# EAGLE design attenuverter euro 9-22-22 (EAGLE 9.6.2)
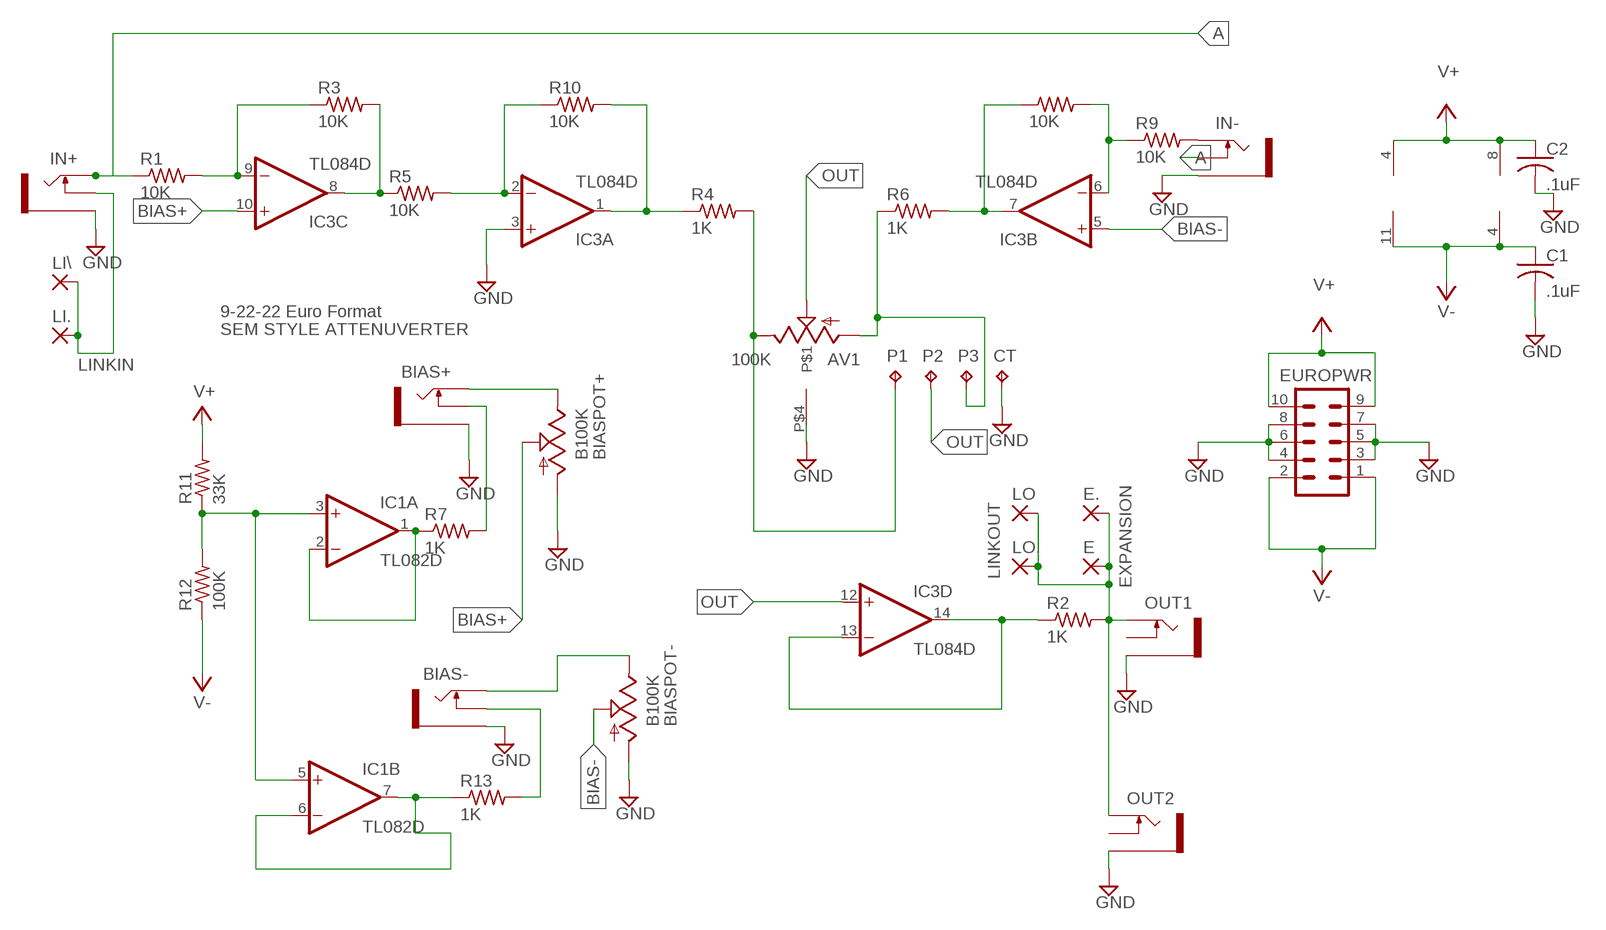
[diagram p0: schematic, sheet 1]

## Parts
AV1  100K  ALPSRK11K114  [ALPSCENTERTAP]
BIAS+  THONKICONNNEW  [WQP-PJ301M-12_JACK]
BIAS-  THONKICONNNEW  [WQP-PJ301M-12_JACK]
BIASPOT+  B100K  9MM_SNAP-IN_POT_  [9MM_SNAP-IN_POT]
BIASPOT-  B100K  9MM_SNAP-IN_POT_  [9MM_SNAP-IN_POT]
C1  .1uF  C-US025-030X050  [C025-030X050]
C2  .1uF  C-US025-030X050  [C025-030X050]
CT  TPPAD1-13  [P1-13]
E  WIREPAD_WIREPAD1,6/0,9  [WIREPAD_1,6/0,9]
E.  WIREPAD_WIREPAD1,6/0,9  [WIREPAD_1,6/0,9]
EUROPWR  EURO_POWER_HEADERREGULAR  [EURO_POWER_HEADER]
IC1  TL082D  [SO08]
IC3  TL084D  [SO14]
IN+  THONKICONNNEW  [WQP-PJ301M-12_JACK]
IN-  THONKICONNNEW  [WQP-PJ301M-12_JACK]
LI.  WIREPAD_WIREPAD1,6/0,9  [WIREPAD_1,6/0,9]
LI\  WIREPAD_WIREPAD1,6/0,9  [WIREPAD_1,6/0,9]
LO  WIREPAD_WIREPAD1,6/0,9  [WIREPAD_1,6/0,9]
LO.  WIREPAD_WIREPAD1,6/0,9  [WIREPAD_1,6/0,9]
OUT1  THONKICONNNEW  [WQP-PJ301M-12_JACK]
OUT2  THONKICONNNEW  [WQP-PJ301M-12_JACK]
P1  TPPAD1-13  [P1-13]
P2  TPPAD1-13  [P1-13]
P3  TPPAD1-13  [P1-13]
R1  10K  R-US_0204/7  [0204/7]
R2  1K  R-US_0204/7  [0204/7]
R3  10K  R-US_0204/7  [0204/7]
R4  1K  R-US_0204/7  [0204/7]
R5  10K  R-US_0204/7  [0204/7]
R6  1K  R-US_0204/7  [0204/7]
R7  1K  R-US_0204/7  [0204/7]
R8  10K  R-US_0204/7  [0204/7]
R9  10K  R-US_0204/7  [0204/7]
R10  10K  R-US_0204/7  [0204/7]
R11  33K  R-US_0204/7  [0204/7]
R12  100K  R-US_0204/7  [0204/7]
R13  1K  R-US_0204/7  [0204/7]

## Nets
A: IN+.P$1_TIP(TIP) IN-.P$2_SWITCH(SWITCH) R1.1
BIAS+: BIASPOT+.2(S) IC3.10(C:+IN)
BIAS-: BIASPOT-.2(S) IC3.5(B:+IN)
GND: AV1.P$4 BIAS+.P$3_SLEEVE(SLEEVE) BIAS-.P$3_SLEEVE(SLEEVE) BIASPOT+.1(A) BIASPOT-.1(A) C1.2 C2.2 CT.TP EUROPWR.3 EUROPWR.4 EUROPWR.5 EUROPWR.6 EUROPWR.7 EUROPWR.8 IC3.3(A:+IN) IN+.P$3_SLEEVE(SLEEVE) IN-.P$3_SLEEVE(SLEEVE) OUT1.P$3_SLEEVE(SLEEVE) OUT2.P$3_SLEEVE(SLEEVE)
N$1: IC3.6(B:-IN) R8.2 R9.1
N$2: IC1.3(A:+IN) IC1.5(B:+IN) R11.1 R12.2
N$3: IC3.7(B:OUT) R6.2 R8.1
N$4: IC1.1(A:OUT) IC1.2(A:-IN) R7.1
N$5: AV1.P$1(HIGH) P1.TP R4.2
N$6: IC1.6(B:-IN) IC1.7(B:OUT) R13.1
N$7: BIAS-.P$1_TIP(TIP) BIASPOT-.3(E)
N$8: IN-.P$1_TIP(TIP) R9.2
N$9: BIAS+.P$2_SWITCH(SWITCH) R7.2
N$10: BIAS-.P$2_SWITCH(SWITCH) R13.2
N$11: IC3.9(C:-IN) R1.2 R3.1
N$12: IC3.13(D:-IN) IC3.14(D:OUT) R2.1
N$13: AV1.P$3(LOW) P3.TP R6.1
N$14: BIAS+.P$1_TIP(TIP) BIASPOT+.3(E)
N$15: E.1(P) E..1(P) LO.1(P) LO..1(P) OUT1.P$1_TIP(TIP) OUT2.P$1_TIP(TIP) R2.2
N$16: IC3.8(C:OUT) R3.2 R5.1
N$17: IC3.2(A:-IN) R5.2 R10.1
N$18: IC3.1(A:OUT) R4.1 R10.2
N$19: IN+.P$2_SWITCH(SWITCH) LI..1(P) LI\.1(P)
OUT: AV1.P$2(WIPER) IC3.12(D:+IN) P2.TP
V+: C2.1 EUROPWR.9 EUROPWR.10 IC1.8(P:V+) IC3.4(P:V+) R11.2
V-: C1.1 EUROPWR.1 EUROPWR.2 IC1.4(P:V-) IC3.11(P:V-) R12.1
Unconnected: OUT1.P$2_SWITCH(SWITCH) OUT2.P$2_SWITCH(SWITCH)

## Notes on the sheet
- 9-22-22 Euro Format
- SEM STYLE ATTENUVERTER
- LINKIN
- LINKOUT
- EXPANSION

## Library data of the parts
AV1 = MusicThingModular-CL:ALPSRK11K114: ALPS Pot with center tap ground
BIAS+ BIAS- IN+ IN- OUT1 OUT2 = MusicThingModular:THONKICONN: 3.5mm socket for Eurorack modular synths
BIASPOT+ BIASPOT- = MusicThingModular:9MM_SNAP-IN_POT: 9mm vertical snap-in pot, Alpha / Panasonic style
C1 C2 = rcl:C-US: CAPACITOR, American symbol; SPICEPREFIX: C
CT P1-P3 = testpad-CL:TP: Test pad NO NAME
E E. LI. LI\ LO LO. = avr328 11-4-21:WIREPAD_WIREPAD: Wire PAD connect wire on PCB
EUROPWR = MusicThingModular:EURO_POWER_HEADER: Power Header 10 pin power header for Eurorack Power Supplies Variants with fatter pads for easier soldering, and the LOCK variant which has 5mil offset pins to hold the component in place before soldering
IC1 = linear:TL082: OP AMP Data sheet; DATA_SHEET: <a href="http://www.ti.com/lit/ds/symlink/tl084a.pdf"> Data sheet </a>
IC3 = linear:TL084: OP AMP
R1-R13 = rcl:R-US_: RESISTOR, American symbol

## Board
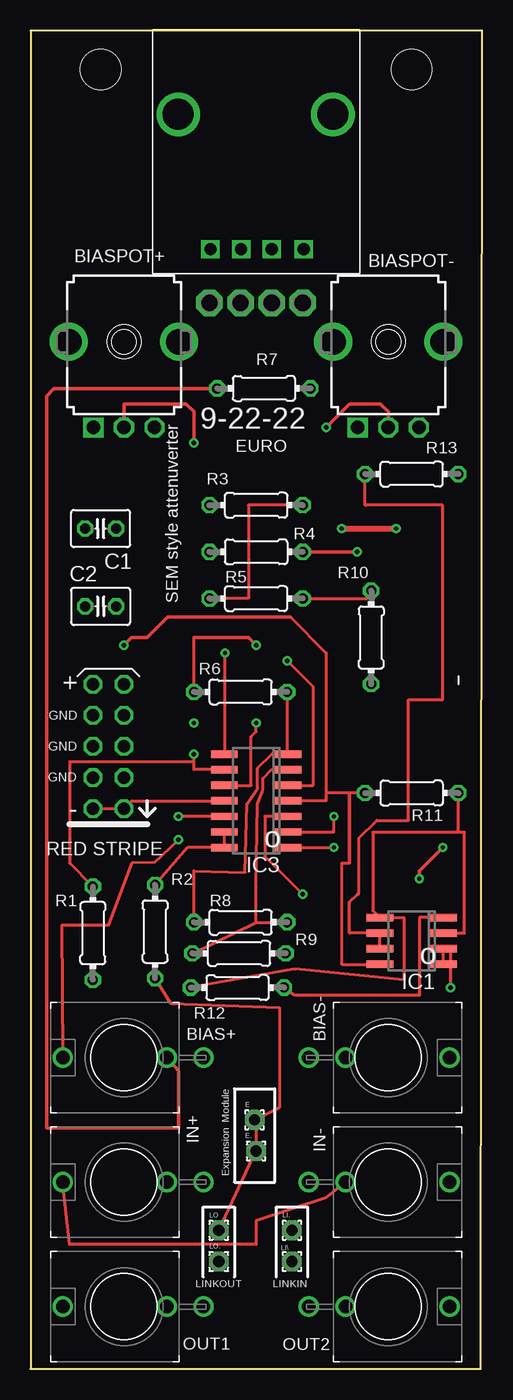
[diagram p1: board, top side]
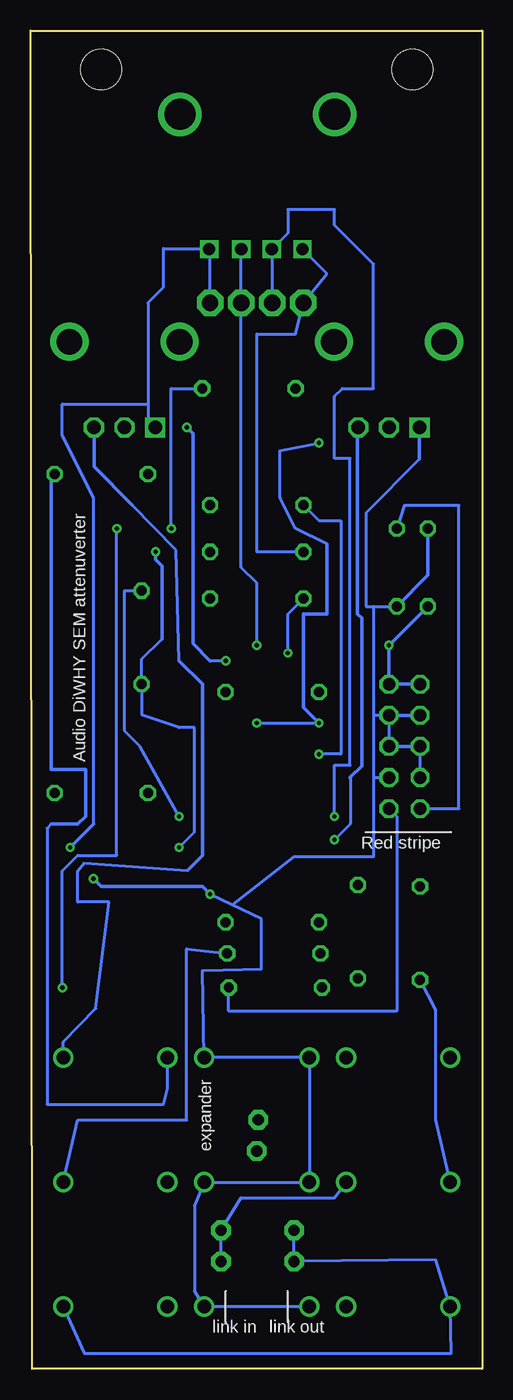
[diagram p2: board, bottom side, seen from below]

Size 36.88 x 109.21 mm. Coordinates in mm from the lower left corner, seen from the top.
Outline: 0,0 36.75,0 36.88,109.21 0,109.21 0,0
Copper layers (1*16): Top 0.035mm / dielectric 1.5mm / Bottom 0.035mm
Design rules "default": minimum track width 6mil, minimum drill 0.35mm, track to track 6mil, track to pad 6mil, pad to pad 6mil, via to via 6mil, smd to smd 6mil, copper to edge 40mil, drill to drill 6mil, minimum pad ring 10mil, minimum via ring 8mil, stop-mask expansion 4mil, vias tented up to drill 0mil, thermal gap 10mil
Holes 3.3 mm at 5.71,106.05 31.11,106.05

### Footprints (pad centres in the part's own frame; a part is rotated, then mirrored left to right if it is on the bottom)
ALPSCENTERTAP = drill 1 square: P$1 10.238,3.746; P$2 12.738,3.746; P$3 15.238,3.746; P$4 17.857,3.746 | drill 2.54: P$5 7.603,14.746; P$6 20.238,14.746
WQP-PJ301M-12_JACK = drill 1.1: P$1_TIP 0,5; P$2_SWITCH 0,-3.5; P$3_SLEEVE 0,-6.5
9MM_SNAP-IN_POT = drill 1.1 square: 1 -2.5,-7 | drill 1.1 octagon: 2 0,-7; 3 2.5,-7 | drill 2.1 pad 2.794: CHASSIS1 -4.5,0; CHASSIS2 4.5,0
C025-030X050 = drill 0.813 octagon: 1 -1.27,0; 2 1.27,0
P1-13 = drill 1.321 pad 2.159 octagon: TP 0,0
WIREPAD_1,6/0,9 = drill 0.914 pad 1.6 octagon: 1 0,0
EURO_POWER_HEADER = drill 1.016 octagon: 1 -5.08,-1.27; 2 -5.08,1.27; 3 -2.54,-1.27; 4 -2.54,1.27; 5 0,-1.27; 6 0,1.27; 7 2.54,-1.27; 8 2.54,1.27; 9 5.08,-1.27; 10 5.08,1.27
SO08 = smd 0.6 x 2.2: 1 -1.905,-2.6; 2 -0.635,-2.6; 3 0.635,-2.6; 4 1.905,-2.6; 5 1.905,2.6; 6 0.635,2.6; 7 -0.635,2.6; 8 -1.905,2.6
SO14 = smd 0.6 x 2.2: 1 -3.81,-2.6; 2 -2.54,-2.6; 3 -1.27,-2.6; 4 0,-2.6; 5 1.27,-2.6; 6 2.54,-2.6; 7 3.81,-2.6; 8 3.81,2.6; 9 2.54,2.6; 10 1.27,2.6; 11 0,2.6; 12 -1.27,2.6; 13 -2.54,2.6; 14 -3.81,2.6
0204/7 = drill 0.813 octagon: 1 -3.81,0; 2 3.81,0

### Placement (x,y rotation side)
AV1  4.45,87.63 0 top
BIAS+  7.62,25.4 90 top
BIAS-  29.21,25.4 270 top
BIASPOT+  7.62,83.82 0 top
BIASPOT-  29.21,83.82 0 top
C1  5.71,68.58 180 top
C2  5.71,62.23 0 top
CT  22.23,87 0 top
E  18.29,20.32 0 top
E.  18.41,17.78 0 top
EUROPWR  6.35,50.8 90 top
IC1  31.11,34.92 90 top
IC3  18.41,46.35 90 top
IN+  7.62,15.24 90 top
IN-  29.21,15.24 270 top
LI.  21.34,11.3 0 top
LI\  21.34,8.76 0 top
LO  15.37,11.3 0 top
LO.  15.37,8.76 0 top
OUT1  7.62,5.08 90 top
OUT2  29.21,5.08 270 top
P1  14.61,87 0 top
P2  17.14,87 0 top
P3  19.68,87 0 top
R1  5.08,35.56 90 top
R2  10.16,35.69 270 top
R3  18.41,70.48 0 top
R4  18.41,66.67 180 top
R5  18.41,62.87 0 top
R6  17.14,55.24 0 top
R7  19.05,80.01 180 top
R8  17.14,36.45 0 top
R9  17.02,33.91 0 top
R10  27.81,59.69 270 top
R11  31.11,46.99 180 top
R12  16.89,31.11 180 top
R13  31.11,73.03 0 top

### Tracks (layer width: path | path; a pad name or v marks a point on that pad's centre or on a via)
A
  Top 0.254: IN-.P$2_SWITCH 24.13,13.97 18.41,12.06 18.41,10.16 3.17,10.16 IN+.P$1_TIP
  Bottom 0.254: R1.1 3.81,29.21 3.81,20.32 IN+.P$1_TIP
BIAS+  (via drill 0.35)
  Top 0.254: IC3.10 18.01,47.62 18.01,51.6 18.41,52.01 v18.41,52.7
  Top 0.305: v13.34,75.56 13.34,78.11 12.7,78.74 7.62,78.74 BIASPOT+.2
  Bottom 0.254: v18.41,52.7 v13.34,52.7 | 12.7,67.31 15.24,68.58 16.51,71.12 16.51,74.93 v13.34,75.56
  Bottom 0.305: v13.34,52.7 14.61,53.98 14.61,61.59 12.7,61.59 12.7,67.31
BIAS-  (via drill 0.35)
  Top 0.254: IC3.5 23.09,47.62 23.09,55.65 v20.95,57.78
  Top 0.305: v24.13,76.83 26.04,78.74 28.57,78.74 29.21,78.11 BIASPOT-.2
  Bottom 0.254: v20.95,57.78 22.23,57.78
  Bottom 0.305: 22.23,57.78 23.62,59.18 23.62,76.33 v24.13,76.83
GND  (via drill 0.35)
  Top 0.254: IC3.3 19.13,45.09 19.13,41.83 v22.23,38.73
  Top 0.305: v31.75,40.01 31.75,40.64 v33.66,42.55
  Bottom 0.152: 22.23,91.3 AV1.P$4
  Bottom 0.254: EUROPWR.5 EUROPWR.7 8.89,53.34 | EUROPWR.6 EUROPWR.4 | 8.89,53.34 8.89,48.26 | 8.89,48.26 EUROPWR.3 | 8.89,62.23 8.89,53.34 | AV1.P$4 25.97,91.38 26.04,91.44 26.04,88.27 27.3,87 27.3,78.74 | CT.TP 22.23,91.3 | 8.89,62.23 9.5,62.23 9.5,69.85 5.12,74.23 | 8.89,62.23 C2.2 | 27.3,78.74 27.3,77.42 BIASPOT-.1 | 8.89,48.26 8.89,41.78 15.4,41.78 20.43,37.87 | BIAS-.P$3_SLEEVE 22.73,25.4 | 22.73,25.4 22.86,32.51 22.73,32.51 18.03,32.64 18.03,36.7 20.43,37.87 | 20.43,37.87 v22.23,38.73 | OUT1.P$3_SLEEVE OUT2.P$3_SLEEVE 23.5,6.35 23.5,13.34 IN-.P$3_SLEEVE IN+.P$3_SLEEVE BIAS+.P$3_SLEEVE 22.73,25.4 | 31.75,44.45 31.75,71.12 34.29,76.2 34.29,78.74 27.3,78.74
  Bottom 0.305: 5.12,74.23 BIASPOT+.1 | v22.23,38.73 22.86,39.37 31.11,39.37 v31.75,40.01 | v33.66,42.55 31.75,44.45 | C2.2 4.45,64.77 C1.2 | EUROPWR.8 EUROPWR.7 | EUROPWR.6 EUROPWR.5
N$1
  Top 0.254: 18.41,36.45 18.41,39.37 18.54,46.1 18.92,47.12 18.92,47.18 18.97,47.23 18.97,48.18 19.68,48.9 IC3.6 | 18.41,36.45 R8.2 | R9.1 18.41,36.45
N$2
  Top 0.254: IC1.3 35.43,35.56 35.43,43.81 34.92,43.81 | 34.92,43.81 R11.1 | 34.92,43.81 27.94,43.81 27.94,37.41 IC1.5 30.48,36.83 30.48,31.75 21.59,32.64 R12.2
N$3
  Top 0.254: IC3.7 20.98,50.2 | 20.98,50.2 20.95,50.23 R6.2 | R8.1 13.34,40.64 17.53,40.51 17.65,46.1 18.54,47.37 18.54,49.02 19.71,50.2 20.98,50.2
N$4  (via drill 0.35)
  Top 0.254: IC1.1 IC1.2 34.29,34.29 v34.29,31.11
  Top 0.508: v25.4,68.58 v29.84,68.58
  Bottom 0.254: R7.1 25.4,80.01 v25.4,68.58 | v34.29,31.11 34.29,40.64 33.02,41.91 29.84,41.91 v29.84,68.58
N$5
  Bottom 0.254: R4.2 18.41,66.67 18.41,84.45 15.24,84.45 P1.TP 12.7,89.39 AV1.P$1
N$6
  Top 0.254: IC1.7 IC1.6 26.04,35.56 26.04,38.1 26.67,38.73 26.8,38.73 26.8,43.31 28.26,44.77 30.86,44.77 30.86,54.61 33.66,54.61 33.66,70.48 27.3,70.48 R13.1
N$7
  Bottom 0.254: BIAS-.P$1_TIP 34.21,26.67 31.57,29.4 30.48,38.1 33.02,38.1 33.02,40.64 32.51,41.27 24.08,40.69 | 24.77,57.78 25.02,66.8 28.57,70.48
  Bottom 0.305: 24.08,40.69 22.86,41.91 22.86,55.88 24.77,57.78 | BIASPOT-.3 31.71,73.62 28.57,70.48
N$8
  Bottom 0.254: R9.2 24.13,34.29 24.13,20.32 33.02,20.32 IN-.P$1_TIP
N$9
  Top 0.254: 1.29,19.68 12.06,19.68
  Top 0.305: R7.2 1.91,80.01 1.29,79.4 1.29,19.68 | 12.06,19.68 12.06,24.34 BIAS+.P$2_SWITCH
N$10
  Bottom 0.254: 35.2,44.45 35.53,44.12 35.53,21.59 26.04,21.59 25.71,22.88 BIAS-.P$2_SWITCH
  Bottom 0.305: R13.2 35.2,72.75 35.2,48.9 32.38,48.9 32.38,45.09 33.02,44.45 35.2,44.45
N$11  (via drill 0.35)
  Top 0.254: IC3.9 13.34,48.9 13.34,49.53 | 13.34,49.53 3.17,49.53 3.17,41.27 R1.2 | 13.34,49.53 v13.34,50.16
  Bottom 0.254: v13.34,50.16 11.56,50.16 11.56,69.22 13.34,69.22 R3.1
N$12
  Top 0.254: IC3.13 IC3.14 12.83,42.55 R2.1
N$13  (via drill 0.35)
  Top 0.254: R6.1 13.34,59.69
  Top 0.305: v18.41,59.05 17.78,59.69 13.34,59.69
  Bottom 0.152: P3.TP AV1.P$3
  Bottom 0.254: v18.41,59.05 18.41,64.14 19.68,65.41 AV1.P$3
N$14  (via drill 0.35)
  Top 0.254: v12.06,43.18 10.1,41.33 8.26,41.27 6.35,36.2 2.54,36.2 BIAS+.P$1_TIP
  Bottom 0.254: 10.77,48.24 10.77,44.47 v12.06,43.18
  Bottom 0.305: 10.77,48.24 10.79,48.26 9.84,49.21 9.84,61.28 10.19,61.62 10.19,76.75 BIASPOT+.3
N$15
  Top 0.254: R2.2 11.43,29.84 20.32,29.49 20.32,21.34 E.1 18.41,20.19 E..1 LO.1
  Bottom 0.254: OUT2.P$1_TIP 32.51,1.27 2.54,1.27 OUT1.P$1_TIP 3.81,8.89 LO..1 LO.1
N$16  (via drill 0.35)
  Top 0.254: R3.2 17.78,70.48 17.78,62.87 R5.1 | IC3.8 15.88,50.23 v15.88,58.42
  Bottom 0.254: R5.1 15.88,61.59 v15.88,58.42
N$17  (via drill 0.35)
  Top 0.254: R5.2 27.5,62.87 R10.1 | IC3.2 24.77,43.81 v24.77,45.09
  Bottom 0.254: v24.77,45.09 27.94,50.8 29.21,52.07 29.21,63.5 R10.1
N$18  (via drill 0.35)
  Top 0.254: IC3.1 v24.77,42.55
  Top 0.305: v26.67,66.67 R4.1
  Bottom 0.254: v24.77,42.55 23.5,43.81 23.5,52.32 24.77,52.32 27.81,53.37 R10.2 27.81,57.91 26.16,59.56
  Bottom 0.305: 26.16,59.56 26.16,65.53 26.67,66.04 v26.67,66.67
N$19
  Bottom 0.254: LI\.1 LI..1 19.68,13.97 12.06,13.97 IN+.P$2_SWITCH
OUT  (via drill 0.35)
  Top 0.254: IC3.12 v12.06,45.09
  Bottom 0.152: 17.18,87.03 P2.TP
  Bottom 0.254: 17.18,87.03 AV1.P$2 15.88,92.68 15.88,94.61 12.06,94.61 12.06,93.34 8.89,90.17 8.89,80.01 11.43,80.01 12.06,79.38 12.06,74.3 10.79,74.3 10.79,49.28 12.06,49.28 v12.06,45.09
V+  (via drill 0.35)
  Top 0.254: R11.2 26.04,46.99 24.13,46.99 | IC3.4 24.13,46.35 24.13,46.99 | 26.04,41.27 25.4,41.27 25.4,33.02 IC1.8 | 21.21,61.34 24.13,58.42 24.13,46.99
  Top 0.305: 26.04,41.27 26.04,46.99 | 21.21,61.34 11.18,61.34 9.53,59.69 8.26,59.69 v7.62,59.05
  Bottom 0.305: C2.1 7.46,59.21 7.62,59.27 v7.62,59.05 EUROPWR.9 EUROPWR.10
V-
  Top 0.254: EUROPWR.2 EUROPWR.1 8.26,46.35 IC3.11 | IC1.4 31.75,36.83 31.75,30.48 21.59,30.48 20.95,30.86 R12.1
  Bottom 0.254: EUROPWR.2 1.91,45.72 1.91,70.48 6.35,70.48 C1.1 | EUROPWR.1 6.99,45.09 6.99,29.21 20.7,29.21 R12.1

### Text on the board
tNames: 9-22-22 | EURO | SEM style attenuverter | o | o | Module | Expansion | LINKOUT | LINKIN
bNames: Audio DiWHY SEM attenuverter | Red stripe | expander | link in | link out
